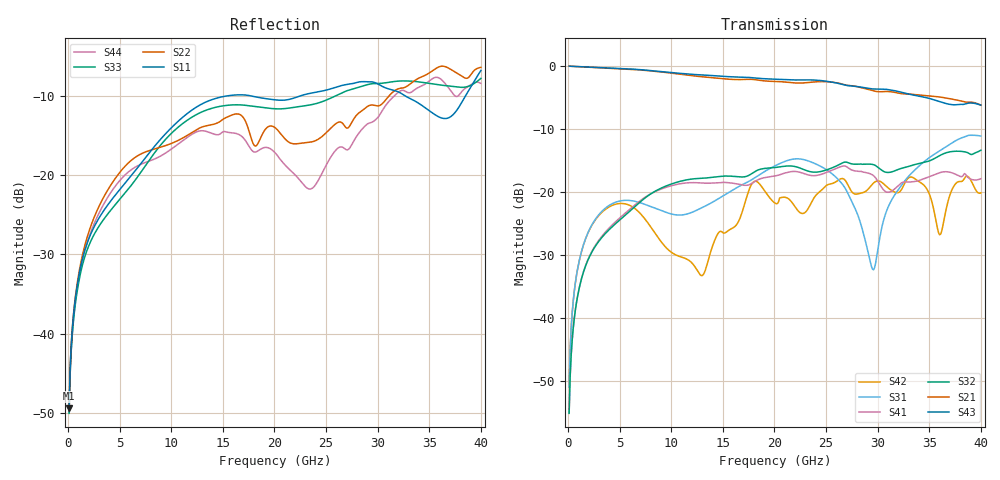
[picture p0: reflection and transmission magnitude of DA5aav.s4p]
! ADC12DJ2700AAV, ADC12DJ3200AAV, ADC08DJ3200AAV
! 144 pin AAV package
! Texas Instruments 4/21/2021
! Single-ended  S-parameters
! PORT#  PORT_NAME  NET_NAME
! PORT1:  DAxN.DIEBUMP DAxN
! PORT2:  DAxN.BGA  DAxN
! PORT3:  DAxP.DIEBUMP DAxP
! PORT4:  DAxP.BGA  DAxP
! Touchstone Ver. 1.0
! Number of ports is 4
# Hz	S	MA	R	50.000000
! SCATTERING PARAMETERS  :
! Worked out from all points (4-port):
!   400 points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, 100 MHz to 40 GHz, reference 50 ohm
!   strongest paths, dB at 100 MHz, 10.1 GHz, 20.1 GHz, 30.1 GHz, 40 GHz:
!     S43: 0.0, -1.0, -2.1, -3.6, -6.2
!     S21: 0.0, -1.1, -2.4, -4.1, -6.2
!     S32: -55.1, -18.7, -16.1, -16.2, -13.3
!     S41: -55.1, -18.9, -17.4, -18.5, -17.9
!     S31: -50.9, -23.5, -15.8, -28.2, -11.1
!     S42: -50.9, -29.6, -21.8, -18.2, -20.1
!   lowest |S11| = -49.4 dB at 100 MHz (marker M1), VSWR 1.01, Z = 50.2 + j0.3 ohm
!   |S11| at or under -10 dB: start of sweep to 15.43 GHz; 17.69 GHz to 22.52 GHz (4.824 GHz wide, 24 % of centre); 32.66 GHz to 38.51 GHz (5.853 GHz wide, 16.4 % of centre)
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1e8  0.003399 61.7  0.9981 -1.3  0.002853 85.0  0.001761 -97.3
     0.9981 -1.3  0.003415 60.5  0.001761 -97.3  0.002851 84.6
     0.002853 85.0  0.001761 -97.3  0.003153 61.7  0.9983 -1.3
     0.001761 -97.3  0.002851 84.6  0.9983 -1.3  0.003168 60.5
9e8  0.02046 68.5  0.9911 -11.3  0.02409 75.7  0.01466 -109.6
     0.9911 -11.3  0.0212 55.4  0.01463 -109.6  0.02399 72.1
     0.02409 75.7  0.01463 -109.6  0.01888 68.6  0.9915 -10.7
     0.01466 -109.6  0.02399 72.1  0.9915 -10.7  0.01963 55.2
3.2e9  0.05639 58.2  0.9686 -39.1  0.06945 48.4  0.04389 -146.5
       0.9686 -39.1  0.06769 9.4  0.04299 -146.0  0.06824 35.4
       0.06945 48.4  0.04299 -146.0  0.04992 60.6  0.9707 -36.9
       0.04389 -146.5  0.06824 35.4  0.9707 -36.9  0.06122 9.1
1.51e10  0.3136 -13.7  0.792 -175.6  0.09421 42.2  0.1196 48.2
         0.792 -175.6  0.2271 -120.7  0.1342 56.5  0.04732 35.8
         0.09421 42.2  0.1342 56.5  0.274 1.5  0.8281 -166.5
         0.1196 48.2  0.04732 35.8  0.8281 -166.5  0.1885 -124.7
2.34e10  0.3274 -58.3  0.7425 92.9  0.1754 -0.7  0.1362 -52.0
         0.7425 92.9  0.1612 95.5  0.1457 -43.5  0.07754 -19.5
         0.1754 -0.7  0.1457 -43.5  0.2768 -37.0  0.777 104.1
         0.1362 -52.0  0.07754 -19.5  0.777 104.1  0.0818 81.8
2.9e10  0.3882 -96.7  0.6575 22.0  0.03535 -19.3  0.1421 -130.0
        0.6575 22.0  0.271 -47.9  0.1669 -106.2  0.1041 176.7
        0.03535 -19.3  0.1669 -106.2  0.3719 -68.8  0.6685 40.2
        0.1421 -130.0  0.1041 176.7  0.6685 40.2  0.2101 -53.7
4e10  0.4569 19.3  0.4897 -115.9  0.2787 -14.6  0.1277 92.9
      0.4897 -115.9  0.4783 -106.4  0.2153 124.9  0.09862 64.3
      0.2787 -14.6  0.2153 124.9  0.4072 110.7  0.4902 -81.4
      0.1277 92.9  0.09862 64.3  0.4902 -81.4  0.3791 -119.9
